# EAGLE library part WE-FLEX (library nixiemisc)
WE-FLEX Flexible Transformer for DC/DC Converter Characteristics Transformer with 6 identical windings 4 sizes with 5 different lengths of air gap each Insulation test voltage 500 VAC Low leakage inductance Operating temperature: –40 ºC to +125 ºC By using different circuits more than 375 transformer solutions and about 125 choke solutions possible. Consequently, quick prototyping possibilities Applications All kind of switching regulators -Flyback converters -Forward converters -Push-pull converters -Step-up/step-down converters -SEPIC converter Details see: http://katalog.we-online.de/en/pbs/WE-FLEX? Updated by Dan Xu 2014-07-07 2014 (C) Wurth Elektronik
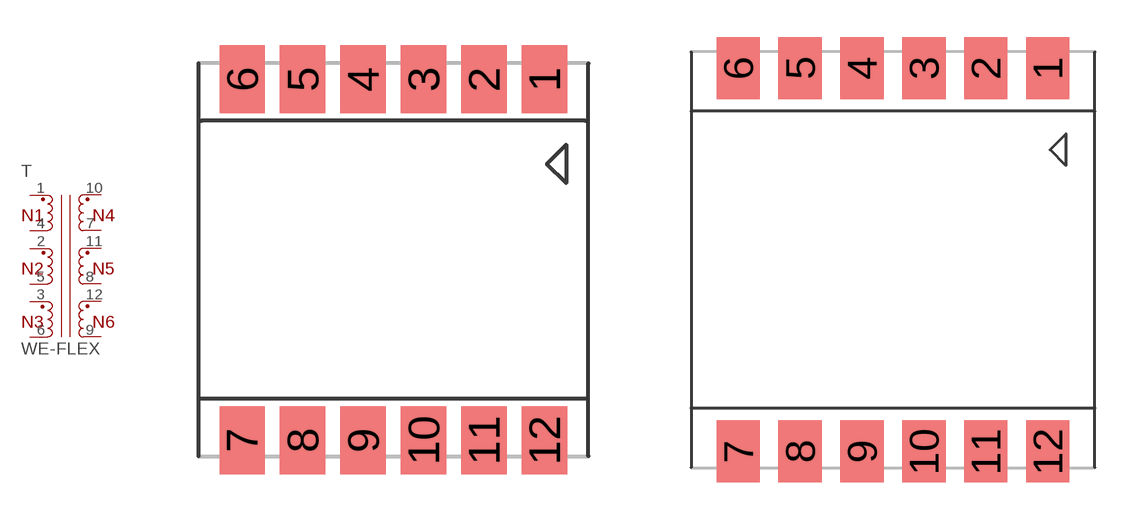
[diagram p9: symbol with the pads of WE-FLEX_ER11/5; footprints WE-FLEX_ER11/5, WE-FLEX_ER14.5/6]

Designator prefix T

## WE-FLEX_ER11/5  [WE-FLEX_ER11/5]
1  1  pas
2  11  pas
3  9  pas
4  12  pas
5  10  pas
6  8  pas
7  3  pas
8  5  pas
9  7  pas
10  2  pas
11  4  pas
12  6  pas

## WE-FLEX_ER14.5/6  [WE-FLEX_ER14.5/6]
1  1  pas
2  11  pas
3  9  pas
4  12  pas
5  10  pas
6  8  pas
7  7  pas
8  5  pas
9  3  pas
10  6  pas
11  4  pas
12  2  pas

## WE-FLEX_EFD15  [WE-FLEX_EFD15]
1  1  pas
2  11  pas
3  9  pas
4  2  pas
5  4  pas
6  6  pas
7  7  pas
8  5  pas
9  3  pas
10  8  pas
11  10  pas
12  12  pas

## WE-FLEX_EFD20  [WE-FLEX_EFD20]
Pads as for WE-FLEX_EFD15

## Footprint WE-FLEX_ER11/5 (pad centres in mm)
smd 1.5 x 2.25: 1 5,5.975; 2 3,5.975; 3 1,5.975; 4 -1,5.975; 5 -3,5.975; 6 -5,5.975; 7 -5,-5.975; 8 -3,-5.975; 9 -1,-5.975; 10 1,-5.975; 11 3,-5.975; 12 5,-5.975

## Footprint WE-FLEX_ER14.5/6 (pad centres in mm)
smd 1.75 x 2.5: 1 6.25,7.75; 2 3.75,7.75; 3 1.25,7.75; 4 -1.25,7.75; 5 -3.75,7.75; 6 -6.25,7.75; 7 -6.25,-7.75; 8 -3.75,-7.75; 9 -1.25,-7.75; 10 1.25,-7.75; 11 3.75,-7.75; 12 6.25,-7.75

## Footprint WE-FLEX_EFD15 (pad centres in mm)
smd 1.75 x 3.43: 1 6.35,10.155; 2 3.81,10.155; 3 1.27,10.155; 4 -1.27,10.155; 5 -3.81,10.155; 6 -6.35,10.155; 7 -6.35,-10.155; 8 -3.81,-10.155; 9 -1.27,-10.155; 10 1.27,-10.155; 11 3.81,-10.155; 12 6.35,-10.155

## Footprint WE-FLEX_EFD20 (pad centres in mm)
smd 2.25 x 3.5: 1 7.5,13.1; 2 4.5,13.1; 3 1.5,13.1; 4 -1.5,13.1; 5 -4.5,13.1; 6 -7.5,13.1; 7 -7.5,-13.1; 8 -4.5,-13.1; 9 -1.5,-13.1; 10 1.5,-13.1; 11 4.5,-13.1; 12 7.5,-13.1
